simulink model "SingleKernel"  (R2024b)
settings: Solver=VariableStepAuto  StartTime=0.0  StopTime=4096*4  RelTol=1e-3
PreLoadFcn:
  | load taps
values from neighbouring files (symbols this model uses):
  S = sum(round(C0))    [NormalizeCoef.m]
undefined symbols (not defined in the file or in its folder): Evaluation, netlist, Platform, VCK190, Versal, vsva2197, xcvc1902
libraries: aieBasic x2, dspsrcs4 x1, dspobslib x1, aieUtilities x1, vmcUtilities x1

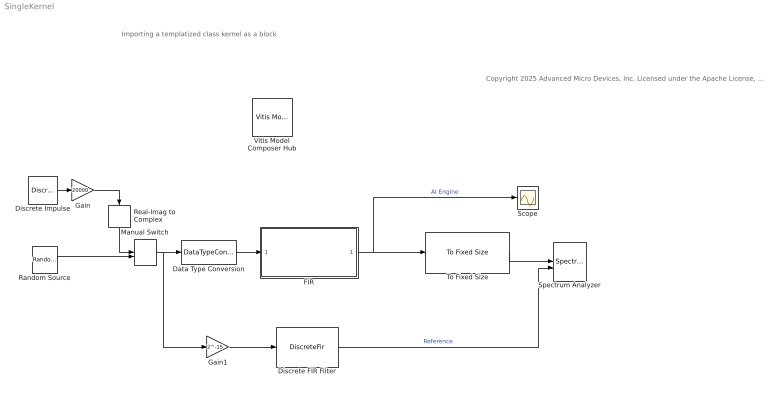
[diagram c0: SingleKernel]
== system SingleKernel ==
  note: Importing a templatized class kernel as a block
  note: Copyright 2025 Advanced Micro Devices, Inc. Licensed under the Apache License, Version 2.0 (the "License"); you may not use this file except in compliance with the License. You may obtain a copy of the License at http://www.apache.org/licenses/LICENSE-2.0 Unless required by applicable law or agreed to in writing, software distributed under the License is distributed on an "AS IS" BASIS, WITHOUT WARRANTIES OR CONDITIONS OF ANY KIND, either express or implied. See the License for the specific language governing permissions and limitations under the License.
  Data Type Conversion : DataTypeConversion  OutDataTypeStr=int16
  Discrete Impulse : dspsrcs4/Discrete  Impulse  Delay=0  SampleTime=1  FrameSample=512  OutputFrames=off  dataType=double  isSigned=on  wordLen=16  udDataType=sfix(16)  fracBitsMode=Best precision  numFracBits=15  OutDataTypeStr=double  LastOutDataTypeStr=double
  Discrete FIR Filter : DiscreteFir  Coefficients=taps'  InputProcessing=Columns as channels (frame based)
  FIR : Subsystem
  Gain : Gain  Gain=20000
  Gain1 : Gain  Gain=2^-15
  Manual Switch : ManualSwitch  CurrentSetting=0
  Random Source : dspobslib/Random Source  SrcType=Uniform  NormMethod=Ziggurat  CltLength=12  MinVal=-20000  MaxVal=20000  MeanVal=0  VarVal=1  RepMode=Not repeatable  rawSeed=1  IsInherit=off  SampMode=Discrete  SampTime=1  SampFrame=512  DataType=Double  OutComplex=Complex  OutputFrames=off
  Real-Imag to Complex : RealImagToComplex  Input=Real
  Scope : Scope
  Spectrum Analyzer : SpectrumAnalyzer  NumInputPorts=2  WindowPosition=[772.000000,1.000000,836.000000,436.000000,]  ScopeFrameLocation=window  Method=Welch  SampleRate=1  Span=1  StartFrequency=-0.5  StopFrequency=0.5  AveragingMethod=Running  YLimits=[-12.103337624215633639,106.2379972844575633]  ShowLegend=on  AllowFFTLengthLessThanSamplesPerUpdate=on
  To Fixed Size : aieUtilities/To Fixed Size  Mode=Stop simulation when input variable-size signal is not full  OutputSize=Inherit: Same as input  CopyMethod=Buffer samples to form output  HasStatusOutput=on
  Vitis Model Composer Hub : vmcUtilities/Vitis Model Composer Hub  Tag=genX  CodeGeneration=off  CompilationType=HDLCompilation  ExportTypeV2=IP Catalog  StartColumn=1  NumberOfColumns=1  TargetDirectory=./netlist  exportDesign=off  analyzeDesign=off  validateDesignOnHw=off  ExportType=AI Engines  IpVendor=xilinx.com  IpLibrary=hls  IpVersion=1.0  IpHWLanguage=Verilog  AieCompilerOptions={}  AieSimulatorOptions={}  CreateTestbench=off  TestbenchStackSize=10  RunRtlSim=off  RunCSim=off  RunAieSim=off  AieSimTimeout=50000  RunAieSimProfiling=off  LaunchVitisAnalyzer=off  PlotOutput=off  RunX86Sim=off  X86SimTimeout=10  GenHwImage=off  GenLibadfXo=off  GenHwValidationCode=off  PlatformType=Not Specified  HwSystemType=Baremetal  HwValidationTarget=hw  ProjDevice=Versal VCK190 Evaluation Platform (xcvc1902-vsva2197-2MP-e-S)  ProjDevicePart=xcvc1902-vsva2197-2MP-e-S  AIEType=AIE  SamplePeriod=-1  ClockFrequency=200  DataPathParallelism=1  xilinxfamily=versalaicore  part=xcvc1902  speed=-2MP-e-S  package=vsva2197  directory=./netlist  testbench=off  incr_netlist=off  synthesis_tool=Vivado  clock_wrapper=Clock Enables  dbl_ovrd=According to Block Masks  dcm_input_clock_period=10  sysclk_period=10  simulink_period=1  eval_field=0  LogFileName=''  NThreads=4
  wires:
  Data Type Conversion/1 -> FIR/1(In1)
  FIR/1(Out1) -> To Fixed Size/1, Scope/1  "AI Engine"
  Manual Switch/1 -> Gain1/1, Data Type Conversion/1
  Random Source/1 -> Manual Switch/2
  Discrete Impulse/1 -> Gain/1
  Real-Imag to Complex/1 -> Manual Switch/1
  Gain/1 -> Real-Imag to Complex/1
  Discrete FIR Filter/1 -> Spectrum Analyzer/2  "Reference"
  Gain1/1 -> Discrete FIR Filter/1
  To Fixed Size/1 -> Spectrum Analyzer/1

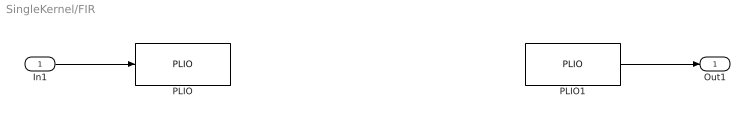
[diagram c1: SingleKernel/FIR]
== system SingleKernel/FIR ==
  In1 : Inport
  PLIO : aieBasic/PLIO  PlioWidth=64  PlioFreqSpec=off  PlioFreq=250  ColLocation=0  channel=0  blockJsonConstraints=[]  deprecateConstraints=0
  PLIO1 : aieBasic/PLIO  PlioWidth=64  PlioFreqSpec=off  PlioFreq=250  ColLocation=0  channel=0  blockJsonConstraints=[]  deprecateConstraints=0
  Out1 : Outport
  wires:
  In1/1 -> PLIO/1
  PLIO1/1 -> Out1/1
